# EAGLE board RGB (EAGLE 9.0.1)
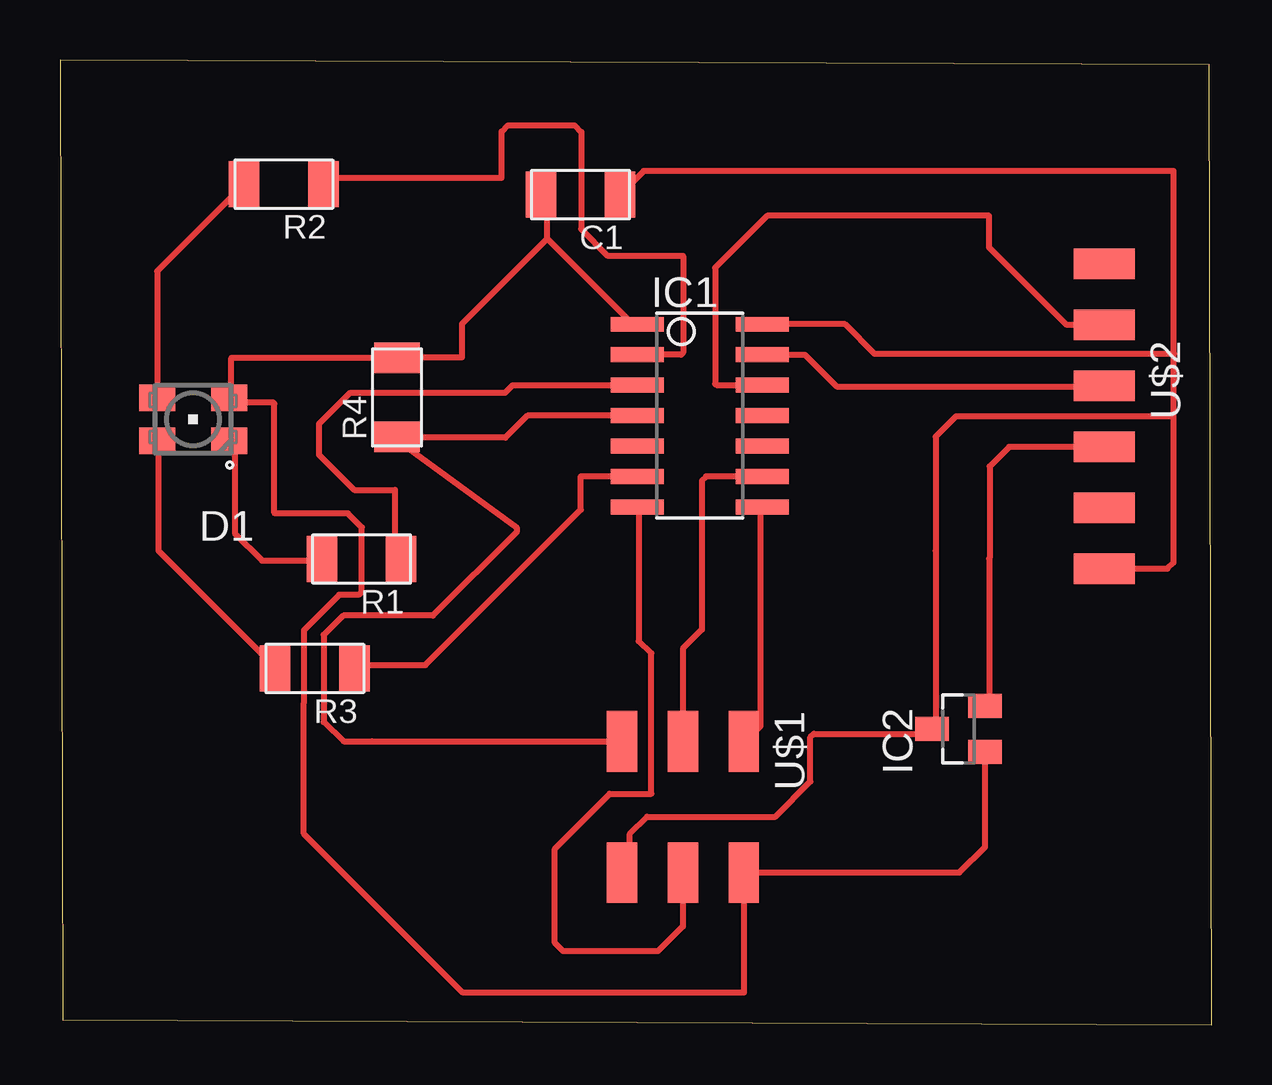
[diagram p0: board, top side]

Size 48 x 40.21 mm. Coordinates in mm from the lower left corner, seen from the top.
Outline: 0.12,0.2 48,0 47.88,40.02 0,40.21 0.12,0.2
Copper layers (1*16): Top 0.035mm / dielectric 1.5mm / Bottom 0.035mm
Design rules "default *": minimum track width 10mil, minimum drill 0.35mm, track to track 12mil, track to pad 12mil, pad to pad 12mil, via to via 12mil, smd to smd 12mil, copper to edge 40mil, drill to drill 6mil, minimum pad ring 10mil, minimum via ring 8mil, stop-mask expansion 4mil, vias tented up to drill 0mil, thermal gap 10mil

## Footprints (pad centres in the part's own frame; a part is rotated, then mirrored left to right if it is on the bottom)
C1206FAB = smd 1.27 x 1.905: 1 -1.651,0; 2 1.651,0
P-LCC-4 = smd 1.1 x 1.5: A 0.902,-1.5; B 0.902,1.5; G -0.902,1.5; R -0.902,-1.5
SOIC14 = smd 0.61 x 2.21: 1 -3.81,-2.603; 2 -2.54,-2.603; 3 -1.27,-2.603; 4 0,-2.603; 5 1.27,-2.603; 6 2.54,-2.603; 7 3.81,-2.603; 8 3.81,2.603; 9 2.54,2.603; 10 1.27,2.603; 11 0,2.603; 12 -1.27,2.603; 13 -2.54,2.603; 14 -3.81,2.603
SOT23 = smd 1 x 1.4: 1 -0.95,-1.1; 2 0.95,-1.1; 3 0,1.1
R1206FAB = smd 1.27 x 1.905: 1 -1.651,0; 2 1.651,0
2X03SMD = smd 2.54 x 1.27: 1 -2.54,2.54; 2 2.92,2.54; 3 -2.54,0; 4 2.92,0; 5 -2.54,-2.54; 6 2.92,-2.54
1X06SMD = smd 2.54 x 1.27: 1 0,6.35; 2 0,3.81; 3 0,1.27; 4 0,-1.27; 5 0,-3.81; 6 0,-6.35

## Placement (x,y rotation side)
C1  1uF  [C1206FAB]  21.69,34.6 180 top
D1  LEDRGBNEW  [P-LCC-4]  5.54,25.24 90 top
IC1  ATTINY44-SSU  [SOIC14]  26.66,25.39 270 top
IC2  5V  [SOT23]  37.44,12.33 90 top
R1  1k  [R1206FAB]  12.56,19.41 180 top
R2  1k  [R1206FAB]  9.32,35.04 180 top
R3  499  [R1206FAB]  10.62,14.85 180 top
R4  10k  [R1206FAB]  14.05,26.15 90 top
U$1  AVRISPSMD  [2X03SMD]  25.95,9.26 270 top
U$2  FTDI-SMD-HEADER  [1X06SMD]  43.52,25.36 180 top

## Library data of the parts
C1 D1 IC1 IC2 R1-R4 U$1 U$2 = fab

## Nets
BLED: D1.G R3.2
BPIN: IC1.6 R3.1
GLED: D1.B R2.2
GND: C1.1 IC1.14 IC2.3 U$1.6 U$2.1
GPIN: IC1.2 R2.1
MISO: IC1.8 U$1.1
MOSI: IC1.7 U$1.4
RLED: D1.R R1.2
RPIN: IC1.3 R1.1
RST: IC1.4 R4.1 U$1.5
RXD: IC1.12 U$2.5
SCK: IC1.9 U$1.3
TXD: IC1.13 U$2.4
VCC: C1.2 D1.A IC1.1 IC2.1 R4.2 U$1.2
VDD: IC2.2 U$2.3

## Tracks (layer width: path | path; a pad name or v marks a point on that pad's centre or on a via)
BLED
  Top 0.254: D1.G 4.11,24.19 4.11,19.75 8.87,14.99 R3.2
BPIN
  Top 0.254: R3.1 12.36,14.99 15.22,14.99 21.71,21.47 21.71,22.87 24.03,22.87 IC1.6 23.79,22.92
GLED
  Top 0.254: 4.11,26.42 D1.B 4.05,31.41 R2.2 7.6,34.99
GND
  Top 0.254: 23.48,6.41 U$1.6 23.75,6.68 23.75,7.96 24.46,8.67 29.8,8.67 31.27,10.14 31.27,11.99 31.41,12.13 36.18,12.13 IC2.3 36.49,12.45 36.49,19.75 36.49,24.52 37.34,25.36 46.39,25.36 46.4,25.35 | 23.48,34.35 C1.1 24.32,35.58 46.4,35.58 46.4,28.01 | 43.8,19.11 U$2.1 46.15,19.01 46.4,19.26 46.4,25.35 | 46.4,25.35 46.4,28.01 | 46.4,28.01 46.42,27.96 33.94,27.96 32.72,29.2 IC1.14
GPIN
  Top 0.254: R2.1 11.09,35.31 18.4,35.31 18.4,37.23 18.66,37.49 21.44,37.49 21.73,37.21 21.73,35.64 21.71,35.63 21.71,33.16 22.83,32.04 25.96,32.04 25.96,28.01 25.88,27.93 IC1.2
MISO
  Top 0.254: IC1.8 29.19,21.34 29.19,12.45 28.56,11.81 U$1.1
MOSI
  Top 0.254: IC1.7 24.11,21.34 24.11,15.99 24.64,15.49 24.64,9.62 22.9,9.62 20.62,7.34 20.62,3.4 20.96,3.06 24.91,3.06 25.95,4.1 U$1.4 25.7,6.1
RLED
  Top 0.254: D1.R 7.28,24.19 7.28,20.48 8.42,19.34 10.85,19.34 R1.2 10.78,19.43
RPIN
  Top 0.254: R1.1 13.95,19.43 13.95,22.29 12.26,22.29 10.8,23.75 10.8,25.05 12.1,26.35 18.55,26.35 18.86,26.66 IC1.3
RST
  Top 0.254: 23.79,25.46 IC1.4 19.47,25.39 18.56,24.47 14.31,24.47 14.27,24.51 R4.1 14.27,24.19 19.05,20.7 19.05,20.57 15.53,17.05 11.81,17.05 10.99,16.25 10.99,12.62 11.81,11.81 13,11.81 23.16,11.81 U$1.5
RXD
  Top 0.254: 29.19,26.73 29.2,26.73 | 29.2,26.73 IC1.12 | 43.48,28.96 U$2.5 41.95,29.17 38.72,32.4 38.72,33.72 29.47,33.72 27.3,31.55 27.3,26.71 27.35,26.67 29.13,26.67 29.2,26.73
SCK
  Top 0.254: 25.7,11.81 U$1.3 25.95,15.68 26.74,16.47 26.74,22.67 26.92,22.85 IC1.9
TXD
  Top 0.254: 43.48,26.73 U$2.4 43.5,26.61 32.36,26.61 31.03,27.93 IC1.13
VCC
  Top 0.254: IC2.1 38.4,11.18 38.55,11.03 38.55,7.41 37.48,6.34 U$1.2 | 28.56,6.41 U$1.2 | 7.28,26.42 D1.A | 13.95,28 R4.2 | 20.3,32.77 20.3,34.04 | 20.3,34.04 20.3,34.35 C1.2 20.3,34.04 | 20.3,32.77 23.79,29.27 IC1.1 | R4.2 14.27,28 14.46,27.81 16.74,27.81 16.74,29.21 20.3,32.77 | 28.24,6.1 U$1.2 | 7.28,26.1 D1.A | U$1.2 28.49,1.35 28.51,1.33 23.48,1.33 16.79,1.33 10.16,7.96 10.16,13.42 10.17,13.43 10.17,16.45 11.63,17.91 12.45,17.91 12.58,18.04 12.58,20.73 11.99,21.32 8.95,21.32 8.94,21.33 8.94,25.89 8.87,25.95 7.23,25.95 D1.A | D1.A 7.14,26.23 7.14,27.79 7.15,27.8 R4.2
VDD
  Top 0.254: IC2.2 38.72,13.4 38.72,19.43 38.74,19.45 38.74,23.28 39.55,24.09 U$2.3 43.48,24.19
